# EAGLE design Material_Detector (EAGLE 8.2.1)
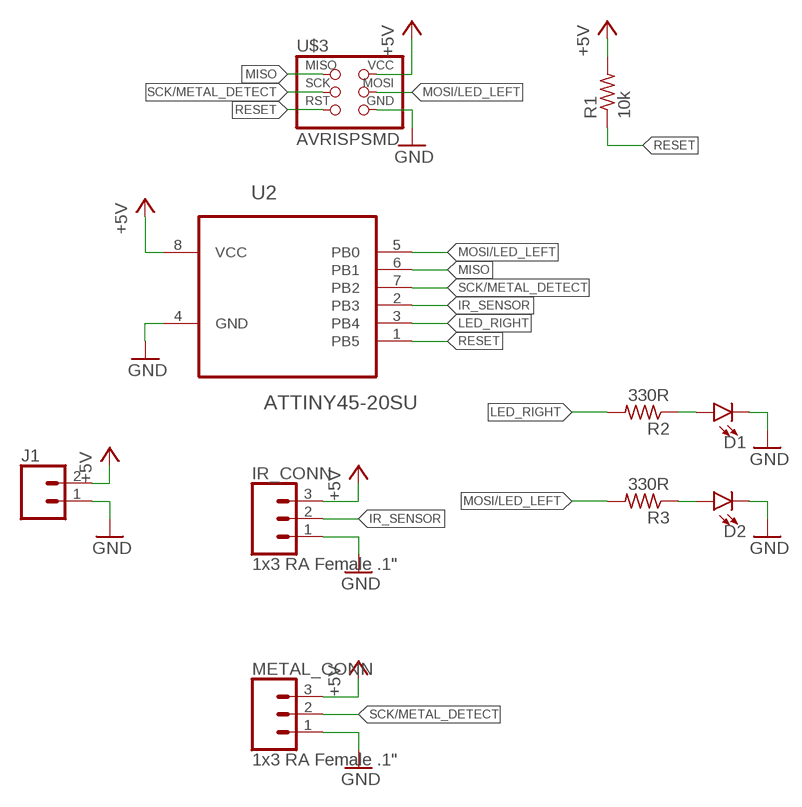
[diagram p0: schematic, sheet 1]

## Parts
D1  LED1206  [LED-1206]
D2  LED1206  [LED-1206]
IR_CONN  1x3 RA Female .1"  CONN_03  [1X03]
J1  CONN_02  [1X02]
METAL_CONN  1x3 RA Female .1"  CONN_03  [1X03]
R1  10k  R-US_R1206  [R1206]
R2  330R  R-US_R1206  [R1206]
R3  330R  R-US_R1206  [R1206]
U2  ATTINY45-20SU  [SOIC127P798X216-8N]
U$3  AVRISPSMD  [2X03SMD]

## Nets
+5V: IR_CONN.3 J1.2 METAL_CONN.3 R1.2 U2.8(VCC) U$3.2(VCC)
GND: D1.C D2.C IR_CONN.1 J1.1 METAL_CONN.1 U2.4(GND) U$3.6(GND)
IR_SENSOR: IR_CONN.2 U2.2(PB3)
LED_RIGHT: R2.2 U2.3(PB4)
MISO: U2.6(PB1) U$3.1(MISO)
MOSI/LED_LEFT: R3.2 U2.5(PB0) U$3.4(MOSI)
N$1: D2.A R3.1
N$4: D1.A R2.1
RESET: R1.1 U2.1(PB5) U$3.5(RST)
SCK/METAL_DETECT: METAL_CONN.2 U2.7(PB2) U$3.3(SCK)

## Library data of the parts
D1 D2 = SparkFun-LED:LED: LED (Generic)
IR_CONN METAL_CONN = SparkFun-Connectors:CONN_03: Multi connection point. Often used as Generic Header-pin footprint for 0.1 inch spaced/style header connections On any of the 0.1 inch spaced packages, you can populate with these: Break Away Headers - Straight (PRT-00116) Break Away Male Headers - Right Angle (PRT-00553) Female Headers (PRT-00115)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
J1 = SparkFun-Connectors:CONN_02: Multi connection point. Often used as Generic Header-pin footprint for 0.1 inch spaced/style header connections
R1-R3 = rcl:R-US_: RESISTOR, American symbol
U2 = Atmel_By_element14_Batch_1-00:ATTINY45-20SU: 8-bit Microcontroller with 4 Bytes In-System Programmable Flash; MPN: ATTINY45-20SU; OC_FARNELL: 1288353; OC_NEWARK: 23M5073; PACKAGE: SOIC-8; SUPPLIER: Atmel
U$3 = fab:AVRISP

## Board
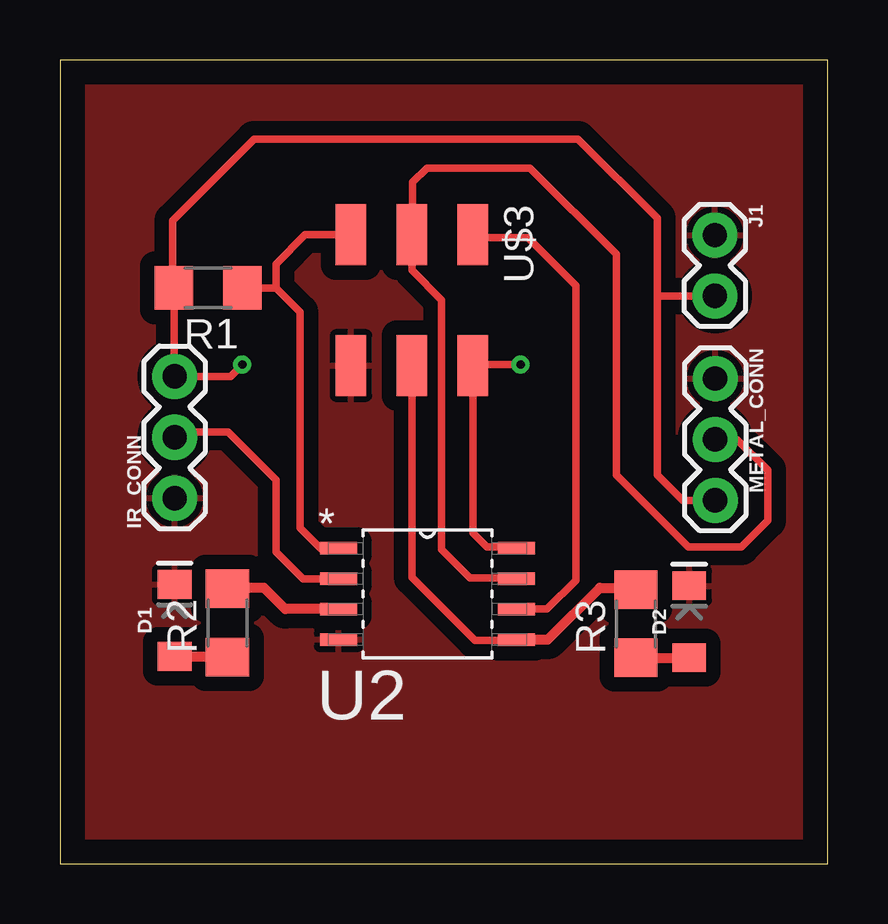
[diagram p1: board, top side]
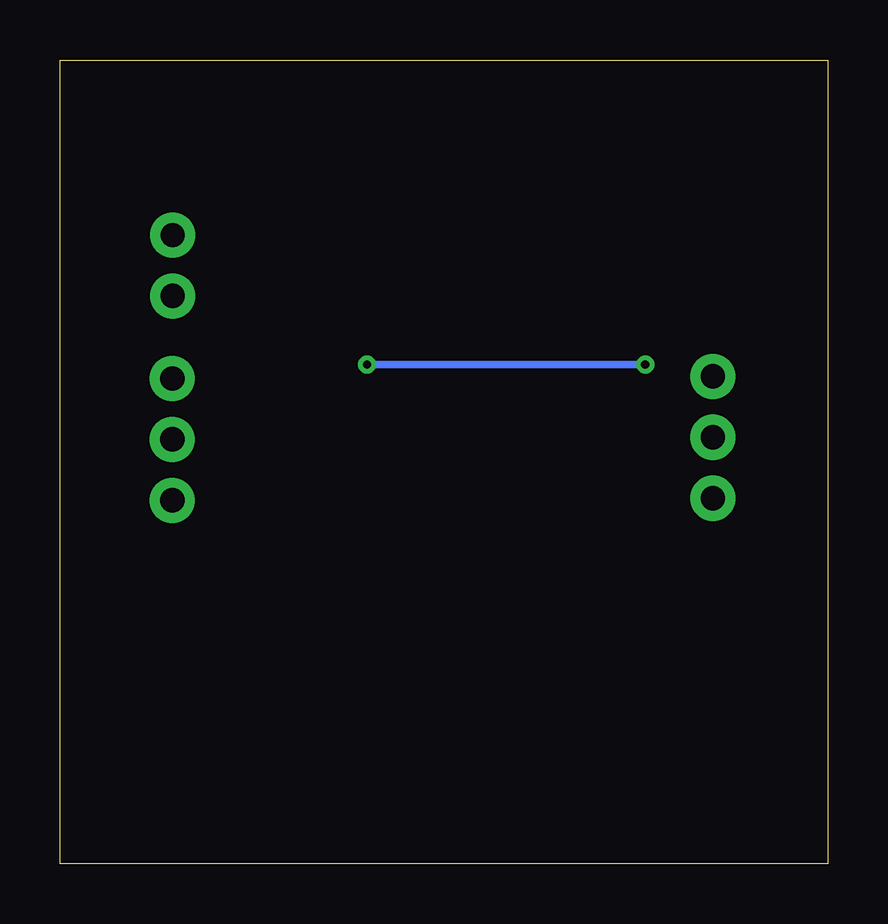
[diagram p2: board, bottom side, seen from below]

Size 32 x 33.5 mm. Coordinates in mm from the lower left corner, seen from the top.
Outline: 0,0 32,0 32,33.5 0,33.5 0,0
Copper layers (1*16): Top 0.035mm / dielectric 1.5mm / Bottom 0.035mm
Design rules "default *": minimum track width 6mil, minimum drill 0.35mm, track to track 0.4mm, track to pad 0.4mm, pad to pad 0.4mm, via to via 0.4mm, smd to smd 6mil, copper to edge 40mil, drill to drill 6mil, minimum pad ring 10mil, minimum via ring 8mil, stop-mask expansion 4mil, vias tented up to drill 0mil, thermal gap 10mil

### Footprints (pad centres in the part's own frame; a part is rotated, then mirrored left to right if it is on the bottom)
LED-1206 = smd 1.2 x 1.4: A -1.5,0; C 1.5,0
1X03 = drill 1.016 pad 1.88: 1 0,0; 2 2.54,0; 3 5.08,0
1X02 = drill 1.016 pad 1.88: 1 0,0; 2 2.54,0
R1206 = smd 1.6 x 1.803: 1 -1.422,0; 2 1.422,0
SOIC127P798X216-8N = smd 1.549 x 0.533: 1 -3.708,1.905; 2 -3.708,0.635; 3 -3.708,-0.635; 4 -3.708,-1.905; 5 3.708,-1.905; 6 3.708,-0.635; 7 3.708,0.635; 8 3.708,1.905
2X03SMD = smd 2.54 x 1.27: 1 -2.54,2.54; 2 2.92,2.54; 3 -2.54,0; 4 2.92,0; 5 -2.54,-2.54; 6 2.92,-2.54

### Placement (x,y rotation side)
D1  4.78,10.13 90 top
D2  26.23,10.08 90 top
IR_CONN  4.78,15.23 90 top
J1  27.3,26.2 270 top
METAL_CONN  27.32,20.22 270 top
R1  6.18,24 180 top
R2  6.98,10.03 90 top
R3  24.01,10 90 top
U2  15.32,11.24 0 top
U$3  14.67,23.68 270 top

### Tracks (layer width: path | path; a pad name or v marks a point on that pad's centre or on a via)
+5V  (via drill 0.35)
  Top 0.305: U2.8 18.97,13.2 17.8,13.2 17.21,13.79 U$3.2 17.25,20.8 v19.2,20.8 | v7.6,20.8 7.11,20.31 IR_CONN.3 4.76,20.33 R1.2 4.7,24.06 4.7,26.8 8.1,30.2 21.6,30.2 24.9,26.9 24.9,23.6 | METAL_CONN.3 25.96,15.14 24.9,16.2 24.9,23.6 | J1.2 24.96,23.66 24.9,23.6
  Bottom 0.305: v7.6,20.8 v19.2,20.8
GND
  pour Top (isolate 0.61): 0,33.5 32,33.5 32,0 0,0
IR_SENSOR
  Top 0.305: U2.2 10.12,11.88 9,13 9,16 7,18 5.01,18 IR_CONN.2
LED_RIGHT
  Top 0.406: U2.3 9.39,10.61 8.5,11.5 7.03,11.5 R2.2
MISO
  Top 0.305: U2.6 20.3,10.61 21.5,11.8 21.5,24.1 19.5,26.1 17.33,26.1 U$3.1
MOSI/LED_LEFT
  Top 0.305: U$3.4 14.67,11.93 17.3,9.3 18.99,9.3 U2.5
  Top 0.406: U2.5 20.34,9.34 22.5,11.5 23.93,11.5 R3.2
N$1
  Top 0.406: R3.1 D2.A
N$4
  Top 0.406: D1.A 6.96,8.63 R2.1
RESET
  Top 0.305: U2.1 10.86,13.14 10,14 10,23 9,24 | 9,24 R1.1 | U$3.5 10.22,26.22 9,25 9,24
SCK/METAL_DETECT
  Top 0.305: U2.7 19,11.9 17.1,11.9 15.9,13.1 15.9,23.5 14.67,24.73 U$3.3 14.7,26.25 14.7,28.4 15.3,29 19.6,29 23.2,25.4 23.2,16.2 26.2,13.2 28.4,13.2 29.5,14.3 29.5,16.4 28.22,17.68 METAL_CONN.2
